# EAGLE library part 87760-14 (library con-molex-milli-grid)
HEADER
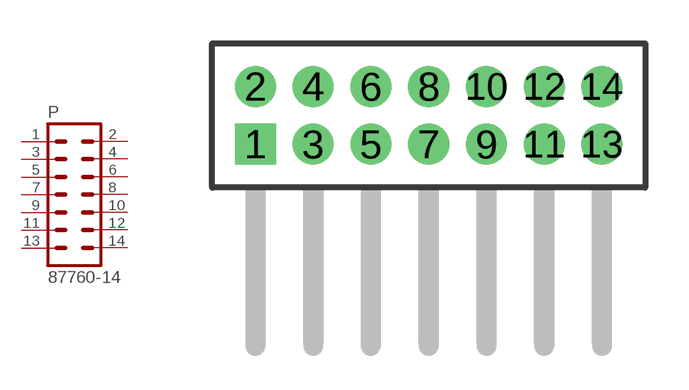
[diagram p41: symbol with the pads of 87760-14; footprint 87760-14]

Designator prefix P

## 87760-14  [87760-14]
1  1  pas
2  2  pas
3  3  pas
4  4  pas
5  5  pas
6  6  pas
7  7  pas
8  8  pas
9  9  pas
10  10  pas
11  11  pas
12  12  pas
13  13  pas
14  14  pas

## Footprint 87760-14 (pad centres in mm)
HEADER Dual Row, Right Angle
drill 0.914 square: 1 -6,-1
drill 0.914: 2 -6,1; 3 -4,-1; 4 -4,1; 5 -2,-1; 6 -2,1; 7 0,-1; 8 0,1; 9 2,-1; 10 2,1; 11 4,-1; 12 4,1; 13 6,-1; 14 6,1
